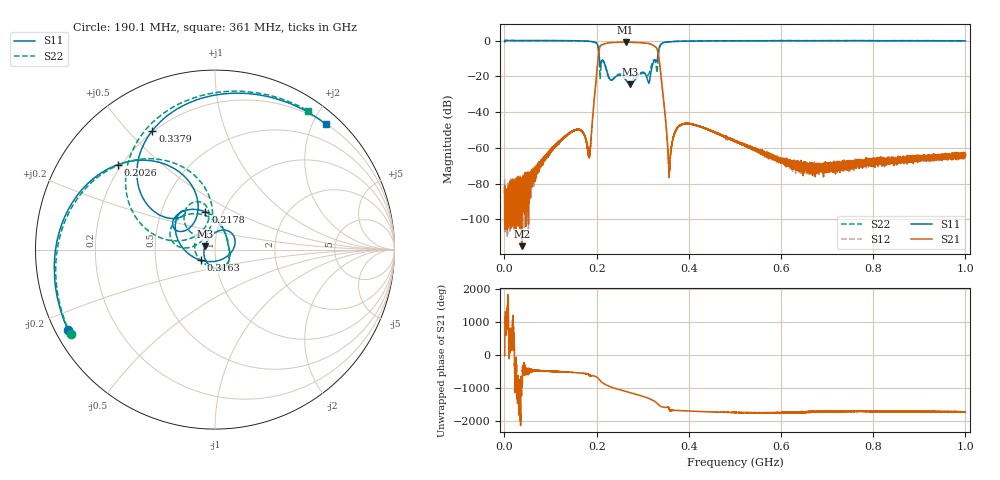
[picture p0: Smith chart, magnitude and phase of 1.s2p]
!Keysight Technologies,N5232A,MY52221221,A.10.65.11
!Date: Thursday, November 09, 2023 14:40:25
!Correction: S11(Full 2 Port(1,4))
!S41(Full 2 Port(1,4))
!S14(Full 2 Port(1,4))
!S44(Full 2 Port(1,4))
!S2P File: Measurements: S11, S41, S14, S44:
# Hz S  RI  R 50
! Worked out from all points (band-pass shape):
!   16001 points, 300 kHz to 1 GHz, reference 50 ohm
!   highest |S21| = -0.94 dB at 262.8 MHz (marker M1); lowest = -115.1 dB at 37.35 MHz (marker M2)
!   |S21| within 3 dB of the highest: 206.4 MHz to 329.4 MHz (123 MHz wide, 45.9 % of centre)
!   lowest |S11| = -24.5 dB at 273.4 MHz (marker M3), VSWR 1.13, Z = 44.6 + j1.64 ohm
!   |S11| at or under -10 dB: 206 MHz to 331.9 MHz (125.9 MHz wide, 46.8 % of centre)
!   |S22| runs from -22.3 to 0.0 dB; largest |S21 - S12| = 0.0022
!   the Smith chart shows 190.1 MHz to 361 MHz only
!   S11 on the Smith chart (normalised r, x): 190.1 MHz: 0.04, -0.26; 202.6 MHz: 0.19, +0.36; 217.8 MHz: 0.83, +0.37; 316.3 MHz: 0.85, -0.10; 337.9 MHz: 0.19, +0.59; 361 MHz: 0.20, +2.21
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300000  1.004 -0.00725  6.04e-05 -1.17e-05  1.97e-05 -0.000132  1.002 -0.00713
3.735138e7  0.9573 -0.2729  4.31e-07 1.71e-06  -2.04e-05 -5.91e-05  0.9586 -0.2679
1.669375e8  -0.2257 -0.9505  -0.0028 0.00102  -0.00284 0.000971  -0.195 -0.9602
1.828077e8  -0.6322 -0.7144  -0.000266 0.000506  -0.000308 0.000586  -0.6103 -0.7349
1.90118e8  -0.8187 -0.4498  0.000478 0.00427  0.000458 0.00436  -0.8043 -0.4708
2.026143e8  -0.5418 0.4733  0.2677 0.0727  0.2674 0.0727  -0.4878 0.4889
2.105494e8  -0.2336 0.1281  -0.2629 -0.6998  -0.2626 -0.7  -0.2403 0.0492
2.177972e8  -0.0533 0.2107  -0.8133 -0.0633  -0.8131 -0.0631  -0.068 0.1944
2.35292e8  0.0811 -0.00826  0.1489 0.8729  0.1489 0.8723  0.0781 -0.0308
2.628462e8  -0.051 -0.0623  0.7378 -0.5111  0.7371 -0.5111  0.00407 -0.1052
2.734055e8  -0.0566 0.0184  0.2378 -0.8619  0.2385 -0.8611  -0.024 -0.0927
2.978982e8  0.078 0.1021  -0.8544 -0.1322  -0.8555 -0.1322  -0.1089 0.0507
3.163302e8  -0.0776 -0.0598  -0.08 0.7991  -0.0789 0.7995  -0.125 0.0892
3.33575e8  -0.3788 0.2526  0.182 -0.3944  0.1813 -0.3939  -0.3397 0.0834
3.379487e8  -0.3491 0.6632  -0.0694 -0.1451  -0.0692 -0.1449  -0.4635 0.5438
3.547561e8  0.4621 0.7944  -0.000662 -0.000358  -0.000649 -0.000351  0.3453 0.8477
3.610043e8  0.6186 0.6984  -0.000319 0.000777  -0.00028 0.000777  0.5196 0.7724
3.890583e8  0.9201 0.2663  -0.0008 0.00455  -0.000846 0.0046  0.885 0.3663
5.0015e8  0.7916 -0.5851  0.000955 0.00118  0.00103 0.0012  0.8412 -0.512
6.667875e8  0.2833 -0.9482  7.43e-05 0.000329  7.12e-05 0.000226  0.3682 -0.9177
8.33425e8  -0.132 -0.9779  2.04e-06 0.000423  4.07e-05 0.000408  -0.0369 -0.9869
1e9  -0.4306 -0.881  0.000298 0.000604  0.000172 0.00049  -0.3411 -0.9246
